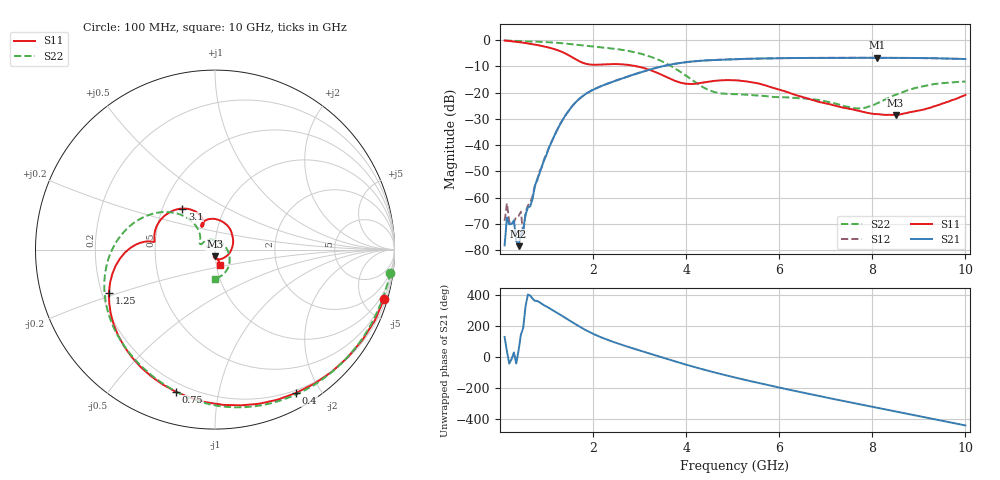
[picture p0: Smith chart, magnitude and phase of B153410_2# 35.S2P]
!  2-Port S-parameters saved by WinCal
! VAR MeasName=S-Parameters (CALIBRATED_DATA) read from VNA (N5245A)
! VAR MeasDate=2016-12-23 10:01:09
! VAR NAME=B153410_2# 35
! VAR FILENAME=B153410_2# 35.S2P
! VAR DATE=2016-12-23 10:01:09
! VAR PHYS_PORTS=1,2
# Hz S DB R 50
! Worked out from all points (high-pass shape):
!   199 points, 100 MHz to 10 GHz, reference 50 ohm
!   highest |S21| = -6.72 dB at 8.1 GHz (marker M1); lowest = -78.5 dB at 400 MHz (marker M2)
!   |S21| within 3 dB of the highest: 3.553 GHz to end of sweep
!   lowest |S11| = -28.5 dB at 8.5 GHz (marker M3), VSWR 1.08, Z = 49.7 - j3.74 ohm
!   |S11| at or under -10 dB: 2.942 GHz to end of sweep
!   |S22| runs from -26.0 to -0.1 dB; largest |S21 - S12| = 0.0023
!   S11 on the Smith chart (normalised r, x): 100 MHz: 0.46, -7.01; 400 MHz: 0.17, -1.70; 750 MHz: 0.15, -0.75; 1.25 GHz: 0.23, -0.19; 3.1 GHz: 0.63, +0.32; 10 GHz: 1.04, -0.18
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1e8  -0.16 -16.2  -78.23 129.5  -68.90 -152.7  -0.13 -7.5
1.5e8  -0.23 -23.9  -67.58 36.1  -62.17 -146.2  -0.17 -10.9
2.5e8  -0.42 -39.0  -70.06 -13.5  -70.27 22.9  -0.25 -17.6
3e8  -0.52 -46.3  -68.69 28.9  -69.54 -58.8  -0.28 -21.0
4e8  -0.75 -60.5  -78.53 42.0  -67.02 -27.4  -0.34 -27.6
4.5e8  -0.86 -67.3  -73.99 144.1  -65.39 -105.0  -0.36 -30.9
5e8  -0.98 -74.0  -72.20 -171.1  -73.89 62.0  -0.39 -34.2
5.5e8  -1.11 -80.6  -66.56 -30.7  -65.54 45.7  -0.43 -37.5
7.5e8  -1.70 -105.3  -55.69 3.7  -55.48 14.7  -0.56 -50.6
1.25e9  -3.90 -157.9  -33.47 -77.9  -33.48 -77.0  -1.05 -82.8
1.75e9  -8.42 173.1  -21.70 -170.5  -21.70 -170.5  -1.97 -112.5
2.45e9  -9.11 159.7  -15.69 95.5  -15.67 95.6  -3.27 -151.0
3.1e9  -10.68 128.5  -11.83 32.6  -11.83 32.4  -5.56 170.9
3.4e9  -12.62 116.4  -10.36 4.5  -10.35 4.4  -7.46 153.6
4.3e9  -16.38 120.5  -7.88 -75.8  -7.89 -76.0  -17.26 130.8
5.05e9  -15.30 93.2  -7.25 -133.8  -7.27 -133.7  -20.60 156.2
5.85e9  -18.08 39.3  -6.94 171.0  -6.95 171.1  -21.61 159.5
6.7e9  -22.76 -31.9  -6.78 116.2  -6.79 116.2  -22.47 145.3
8.1e9  -28.19 -99.8  -6.72 30.3  -6.73 30.3  -24.15 10.3
8.35e9  -28.46 -95.6  -6.76 15.1  -6.74 15.2  -21.98 -14.7
8.5e9  -28.51 -92.0  -6.76 6.2  -6.75 6.1  -20.88 -26.4
1e10  -20.86 -71.2  -7.19 -84.7  -7.21 -84.4  -15.79 -90.7
